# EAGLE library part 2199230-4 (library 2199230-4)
AMP - TE CONNECTIVITY - 2199230-4 - CONNECTOR, CARD EDGE, RCPT, 67POS, 2ROW Source: Datasheet
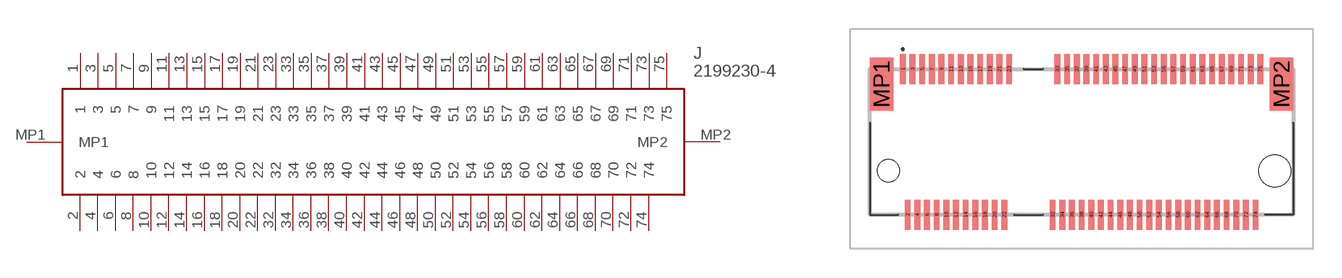
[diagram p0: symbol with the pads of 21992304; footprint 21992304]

Designator prefix J

## 2199230-4 (Description: AMP - TE CONNECTIVITY - 2199230-4 - CONNECTOR, CARD EDGE, RCPT, 67POS, 2ROW; Height: 4.2mm; Manufacturer_Name: TE Connectivity; Manufacturer_Part_Number: 2199230-4; Mouser_Part_Number: 571-2199230-4; Mouser_Price-Stock: https://www.mouser.co.uk/ProductDetail/TE-Connectivity/2199230-4?qs=EQCnRgr4b6HnhitEoflgGQ%3D%3D)  [21992304]
1  1
2  2
3  3
4  4
5  5
6  6
7  7
8  8
9  9
10  10
11  11
12  12
13  13
14  14
15  15
16  16
17  17
18  18
19  19
20  20
21  21
22  22
23  23
32  32
33  33
34  34
35  35
36  36
37  37
38  38
39  39
40  40
41  41
42  42
43  43
44  44
45  45
46  46
47  47
48  48
49  49
50  50
51  51
52  52
53  53
54  54
55  55
56  56
57  57
58  58
59  59
60  60
61  61
62  62
63  63
64  64
65  65
66  66
67  67
68  68
69  69
70  70
71  71
72  72
73  73
74  74
75  75
MP1  MP1
MP2  MP2

## Footprint 21992304 (pad centres in mm)
2199230-4_1
smd 0.3 x 1.55: 1 -9.25,3.625; 2 -9,-3.925; 3 -8.75,3.625; 4 -8.5,-3.925; 5 -8.25,3.625; 6 -8,-3.925; 7 -7.75,3.625; 8 -7.5,-3.925; 9 -7.25,3.625; 10 -7,-3.925; 11 -6.75,3.625; 12 -6.5,-3.925; 13 -6.25,3.625; 14 -6,-3.925; 15 -5.75,3.625; 16 -5.5,-3.925; 17 -5.25,3.625; 18 -5,-3.925; 19 -4.75,3.625; 20 -4.5,-3.925; 21 -4.25,3.625; 22 -4,-3.925; 23 -3.75,3.625; 32 -1.5,-3.925; 33 -1.25,3.625; 34 -1,-3.925; 35 -0.75,3.625; 36 -0.5,-3.925; 37 -0.25,3.625; 38 0,-3.925; 39 0.25,3.625; 40 0.5,-3.925; 41 0.75,3.625; 42 1,-3.925; 43 1.25,3.625; 44 1.5,-3.925; 45 1.75,3.625; 46 2,-3.925; 47 2.25,3.625; 48 2.5,-3.925; 49 2.75,3.625; 50 3,-3.925; 51 3.25,3.625; 52 3.5,-3.925; 53 3.75,3.625; 54 4,-3.925; 55 4.25,3.625; 56 4.5,-3.925; 57 4.75,3.625; 58 5,-3.925; 59 5.25,3.625; 60 5.5,-3.925; 61 5.75,3.625; 62 6,-3.925; 63 6.25,3.625; 64 6.5,-3.925; 65 6.75,3.625; 66 7,-3.925; 67 7.25,3.625; 68 7.5,-3.925; 69 7.75,3.625; 70 8,-3.925; 71 8.25,3.625; 72 8.5,-3.925; 73 8.75,3.625; 74 9,-3.925; 75 9.25,3.625
smd 1.2 x 2.75: MP1 -10.35,2.85; MP2 10.35,2.85
hole 1.15 at -10,-1.65
hole 1.65 at 10,-1.65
